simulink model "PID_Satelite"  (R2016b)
settings: Solver=ode45  StartTime=0.0  StopTime=500  RelTol=1e-3  EnableMultiTasking=on

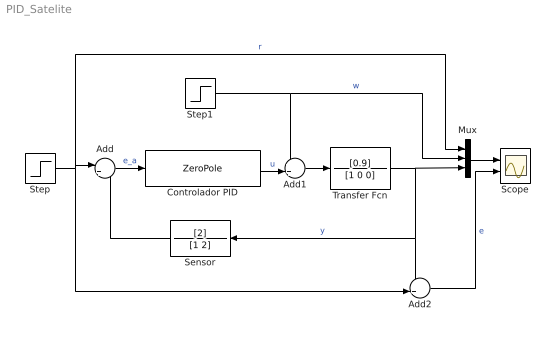
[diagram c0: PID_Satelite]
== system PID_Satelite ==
  Add : Sum  Inputs=|+-
  Add1 : Sum  Inputs=++|
  Add2 : Sum  Inputs=-+|
  Controlador PID : ZeroPole  Zeros=[-0.1 -0.005]  Poles=[0 -100]  Gain=50
  Mux : Mux  Inputs=3
  Scope : Scope  NumInputPorts=2
  Sensor : TransferFcn  Numerator=[2]  Denominator=[1 2]
  Step : Step  Time=0  SampleTime=0
  Step1 : Step  Time=40  After=0  SampleTime=0
  Transfer Fcn : TransferFcn  Numerator=[0.9]  Denominator=[1 0 0]
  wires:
  Step/1 -> Mux/1, Add2/2, Add/1  "r"
  Transfer Fcn/1 -> Add2/1, Sensor/1, Mux/3  "y"
  Add/1 -> Controlador PID/1  "e_a"
  Mux/1 -> Scope/1
  Add2/1 -> Scope/2  "e"
  Sensor/1 -> Add/2
  Add1/1 -> Transfer Fcn/1
  Controlador PID/1 -> Add1/2  "u"
  Step1/1 -> Add1/1, Mux/2  "w"
